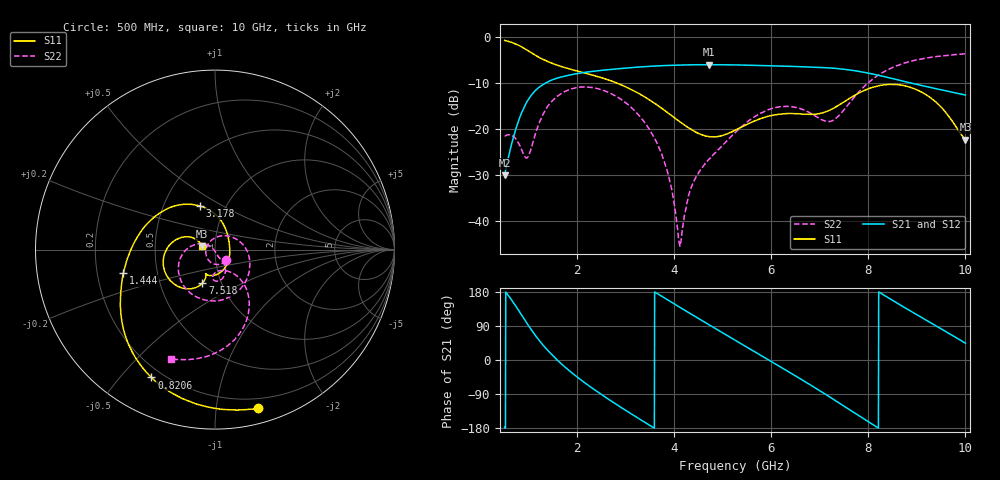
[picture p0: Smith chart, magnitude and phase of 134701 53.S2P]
!  2-Port S-parameters saved by WinCal
! VAR MeasName=S-Parameters (CALIBRATED_DATA) read from VNA (N5242A)
! VAR MeasDate=2013-7-3 16:39:54
! VAR NAME=134701 53
! VAR FILENAME=134701 53.S2P
! VAR DATE=2013-7-3 16:39:54
! VAR PHYS_PORTS=1,2
# Hz S MA R 50
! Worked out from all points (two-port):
!   1601 points, 500 MHz to 10 GHz, reference 50 ohm
!   highest |S21| = -6.02 dB at 4.71 GHz (marker M1); lowest = -30.0 dB at 500 MHz (marker M2)
!   |S21| within 3 dB of the highest: 1.561 GHz to 8.488 GHz (6.927 GHz wide, 138 % of centre)
!   lowest |S11| = -22.3 dB at 10 GHz (marker M3), VSWR 1.17, Z = 43 + j1.64 ohm
!   |S11| at or under -10 dB: 2.812 GHz to end of sweep
!   |S22| runs from -45.4 to -3.7 dB; largest |S21 - S12| = 0.0029
!   S11 on the Smith chart (normalised r, x): 500 MHz: 0.12, -1.30; 820.6 MHz: 0.16, -0.61; 1.444 GHz: 0.31, -0.11; 3.178 GHz: 0.75, +0.39; 7.518 GHz: 0.81, -0.32; 10 GHz: 0.86, +0.03
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5e8  0.9163 -74.7  0.03159 -177.3  0.03162 -177.4  0.08381 -44.6
8.20625e8  0.7956 -116.4  0.1372 124.7  0.1371 124.5  0.06484 -131.3
9.86875e8  0.7053 -134.0  0.2085 91.8  0.2083 91.7  0.05056 132.8
1.444062e9  0.5267 -165.8  0.336 18.0  0.3358 17.9  0.1925 -11.0
1.740938e9  0.4651 179.1  0.3765 -18.2  0.376 -18.3  0.2556 -53.4
2.085312e9  0.4151 162.8  0.408 -53.7  0.4073 -53.8  0.2865 -92.2
2.61375e9  0.3458 137.8  0.4399 -101.2  0.4392 -101.2  0.2537 -139.6
3.177812e9  0.2578 109.3  0.4673 -147.4  0.4663 -147.4  0.1586 179.6
3.670625e9  0.1784 83.1  0.4862 173.5  0.4852 173.6  0.06499 152.6
3.914062e9  0.1437 69.6  0.4916 154.5  0.4918 154.5  0.02602 147.8
4.11e9  0.1206 57.9  0.4949 139.3  0.4946 139.3  0.005501 -145.7
4.3475e9  0.09934 41.5  0.4983 121.0  0.4982 121.1  0.02337 -70.7
4.709688e9  0.08258 10.3  0.5002 93.4  0.4996 93.4  0.04693 -63.4
5.25e9  0.09686 -39.1  0.4971 52.4  0.4974 52.4  0.09124 -57.5
6.021875e9  0.141 -89.0  0.486 -5.8  0.4858 -5.9  0.168 -76.8
6.835312e9  0.1443 -111.3  0.4715 -68.2  0.4716 -68.2  0.1458 -94.7
7.203438e9  0.1602 -108.8  0.4613 -97.6  0.4608 -97.7  0.1211 -75.4
7.518125e9  0.2003 -110.7  0.4447 -123.5  0.4459 -123.6  0.1667 -52.6
7.9575e9  0.2685 -125.5  0.4085 -159.6  0.4094 -159.8  0.3054 -53.2
8.420625e9  0.3051 -149.3  0.3612 163.4  0.3608 163.0  0.4464 -68.0
9.257812e9  0.2234 165.5  0.2847 100.3  0.2837 100.1  0.5969 -94.7
1e10  0.07681 165.7  0.2342 44.4  0.233 44.2  0.6563 -111.9
